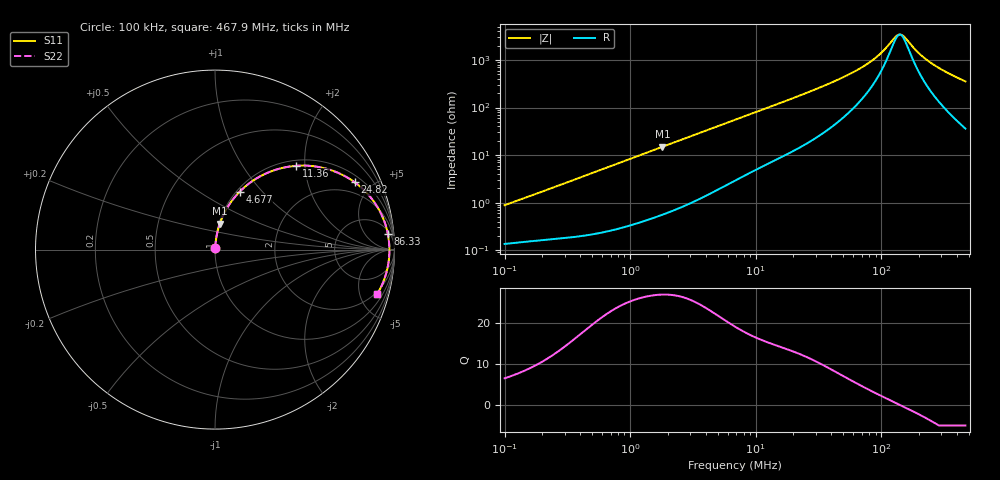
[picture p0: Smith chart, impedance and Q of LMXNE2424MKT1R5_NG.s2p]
! LMXNE2424MKT1R5_NG  S-PARAMETER MODEL  ( General Type )
! Model Generated by TAIYO YUDEN Corporation (https://www.yuden.co.jp/en/)
! Version 1.0
! TAIYO YUDEN Control No. 191023NI43SB-FBB
! Copyright(c) 2019 TAIYO YUDEN CO.,LTD. All Rights Reserved.
! Product Description (link to TY-COMPAS)
! https://ds.yuden.co.jp/TYCOMPAS/or/detail?pn=LMXNE2424MKT1R5NNG&u=M
! Products Name : Inductors
! Characteristics :
!  Inductance : 1.5 uH , SRF(min) : 89 MHz , DC Resistance(max) : 0.12 Ohm
!  Rated Current : Saturation :2100 mA , Temp Rise : 1150 mA (40 degC)
!  Case Size : 2.4 x 2.4 / 0.095 x 0.095 [mm/inch] , Thickness : 1.2 / 0.047 [mm/inch]
!  (Conditions: Temperature = 25 degC , DC Bias Current/Voltage = 0A / 0V)
! External Node Assignments :
!  1  o---GGG---o  2
! GND o---------o GND
! Frequency Range : 0.1MHz  -  467.920999MHz  [ 402 STEP ]
# MHz S RI R 50
! Freq[MHz].  S11 Real  S11 Imag  S21 Real  S21 Imag  S12 Real  S12 Imag  S22 Real  S22 Imag
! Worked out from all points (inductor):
!   401 points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, 100 kHz to 467.9 MHz, reference 50 ohm
!   read as one part in series: L = 1.37 uH near 104.3 kHz
!   highest Q = 26.8 at 1.807 MHz (marker M1), where L = 1.31 uH
!   self-resonance near 140.6 MHz
!   S11 on the Smith chart (normalised r, x): 100 kHz: 1.00, +0.02; 4.677 MHz: 1.03, +0.76; 11.36 MHz: 1.12, +1.81; 24.82 MHz: 1.34, +3.95; 86.33 MHz: 7, +19; 467.9 MHz: 1.72, -7.05
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0.1  0.00143 0.0087  0.9986 -0.0087  0.9986 -0.0087  0.00143 0.0087
0.411864  0.00317 0.0344  0.9968 -0.0344  0.9968 -0.0344  0.00317 0.0344
1.69632  0.0241 0.1359  0.9759 -0.1359  0.9759 -0.1359  0.0241 0.1359
1.807316  0.0269 0.1442  0.9731 -0.1442  0.9731 -0.1442  0.0269 0.1442
3.064925  0.0673 0.2316  0.9327 -0.2316  0.9327 -0.2316  0.0673 0.2316
4.676581  0.1372 0.3223  0.8628 -0.3223  0.8628 -0.3223  0.1372 0.3223
6.986533  0.2522 0.4085  0.7478 -0.4085  0.7478 -0.4085  0.2522 0.4085
11.35786  0.4533 0.4669  0.5467 -0.4669  0.5467 -0.4669  0.4533 0.4669
16.26593  0.6164 0.4517  0.3836 -0.4517  0.3836 -0.4517  0.6164 0.4517
24.81919  0.778 0.3753  0.222 -0.3753  0.222 -0.3753  0.778 0.3753
28.17346  0.8155 0.3451  0.1845 -0.3451  0.1845 -0.3451  0.8155 0.3451
54.23486  0.9325 0.1844  0.0675 -0.1844  0.0675 -0.1844  0.9325 0.1844
69.88496  0.9526 0.1296  0.0474 -0.1296  0.0474 -0.1296  0.9526 0.1296
86.32529  0.9629 0.0879  0.0371 -0.0879  0.0371 -0.0879  0.9629 0.0879
100.0843  0.9675 0.0604  0.0325 -0.0604  0.0325 -0.0604  0.9675 0.0604
116.0364  0.9703 0.0338  0.0297 -0.0338  0.0297 -0.0338  0.9703 0.0338
134.5309  0.9716 0.00773  0.0284 -0.00773  0.0284 -0.00773  0.9716 0.00773
146.3942  0.9717 -0.00707  0.0283 0.00707  0.0283 0.00707  0.9717 -0.00707
196.7795  0.9683 -0.0598  0.0317 0.0598  0.0317 0.0598  0.9683 -0.0598
243.0716  0.9617 -0.0997  0.0383 0.0997  0.0383 0.0997  0.9617 -0.0997
333.7072  0.9429 -0.1659  0.0571 0.1659  0.0571 0.1659  0.9429 -0.1659
467.921  0.9047 -0.247  0.0953 0.247  0.0953 0.247  0.9047 -0.247
